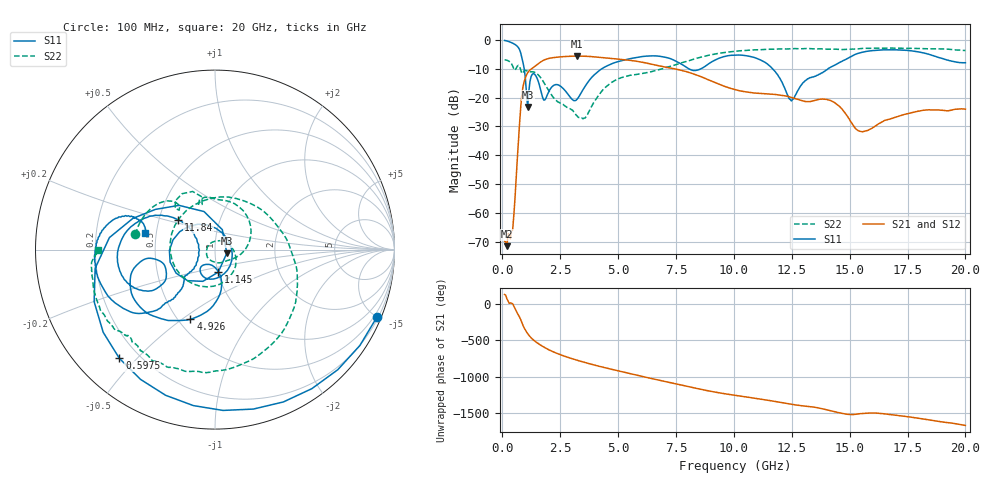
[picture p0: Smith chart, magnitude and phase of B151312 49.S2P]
!  2-Port S-parameters saved by WinCal
! VAR MeasName=S-Parameters (CALIBRATED_DATA) read from VNA (N5244A)
! VAR MeasDate=12/8/2015 5:47:40 PM
! VAR NAME=B151312 49
! VAR FILENAME=B151312 49.S2P
! VAR DATE=12/8/2015 5:47:40 PM
! VAR PHYS_PORTS=1,2
# Hz S DB R 50
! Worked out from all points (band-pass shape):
!   401 points, 100 MHz to 20 GHz, reference 50 ohm
!   highest |S21| = -5.62 dB at 3.234 GHz (marker M1); lowest = -71.6 dB at 199.5 MHz (marker M2)
!   |S21| within 3 dB of the highest: 1.495 GHz to 6.537 GHz (5.043 GHz wide, 126 % of centre)
!   lowest |S11| = -23.2 dB at 1.095 GHz (marker M3), VSWR 1.15, Z = 57 - j2.26 ohm
!   |S11| at or under -10 dB: 946.3 MHz to 4.301 GHz (3.354 GHz wide, 128 % of centre); 8.049 GHz to 8.584 GHz (535.3 MHz wide, 6.44 % of centre); 11.67 GHz to 14.07 GHz (2.397 GHz wide, 18.6 % of centre)
!   |S22| runs from -27.4 to -2.8 dB; largest |S21 - S12| = 0.002
!   S11 on the Smith chart (normalised r, x): 100 MHz: 0.30, -4.99; 597.5 MHz: 0.13, -0.45; 1.145 GHz: 1.00, -0.26; 4.926 GHz: 0.58, -0.54; 11.84 GHz: 0.63, +0.22; 20 GHz: 0.43, +0.09
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1e8  -0.20 -22.6  -69.89 127.5  -70.36 128.7  -6.90 169.3
1.995e8  -0.38 -44.4  -71.58 67.7  -75.02 59.5  -7.08 158.2
4.4825e8  -1.14 -97.9  -65.92 1.0  -65.43 -7.2  -9.08 130.1
5.975e8  -1.86 -131.3  -48.12 -96.1  -48.15 -96.0  -9.92 134.0
8.4625e8  -6.20 159.2  -18.88 103.0  -18.88 103.0  -11.64 105.9
1.095e9  -23.25 -16.6  -11.40 -47.5  -11.40 -47.5  -10.94 91.1
1.14475e9  -17.92 -81.8  -10.87 -68.6  -10.86 -68.6  -11.06 87.4
1.5925e9  -15.40 123.6  -8.02 168.3  -8.02 168.3  -12.48 33.6
2.09e9  -16.83 -69.3  -6.30 79.4  -6.29 79.4  -18.70 -24.5
2.63725e9  -16.94 -125.7  -5.81 9.4  -5.81 9.4  -22.45 -77.9
3.23425e9  -20.54 -94.4  -5.62 -51.7  -5.62 -51.7  -26.39 -171.9
3.43325e9  -17.97 -81.1  -5.64 -70.1  -5.64 -70.1  -27.10 139.5
4.92575e9  -7.71 -109.4  -6.61 169.4  -6.60 169.4  -13.81 -91.9
6.7665e9  -5.65 -153.9  -8.99 36.1  -8.98 36.0  -10.34 71.5
8.20925e9  -10.55 -164.1  -11.69 -64.9  -11.66 -65.0  -6.81 -10.4
1.005e10  -5.25 -170.0  -17.26 -171.4  -17.23 -171.7  -3.95 -66.8
1.1841e10  -11.62 140.8  -18.99 101.0  -19.02 100.8  -3.19 -101.3
1.248775e10  -21.20 -178.5  -19.97 65.9  -20.00 65.8  -3.08 -110.8
1.338325e10  -12.89 -138.4  -21.26 30.3  -21.26 30.2  -3.10 -121.9
1.547275e10  -4.45 -146.1  -31.78 -62.1  -31.76 -62.1  -3.02 -140.3
1.67165e10  -3.46 -171.6  -27.54 -72.8  -27.46 -73.3  -2.83 -151.8
2e10  -7.92 166.8  -24.07 136.3  -24.16 135.8  -3.69 -179.6
